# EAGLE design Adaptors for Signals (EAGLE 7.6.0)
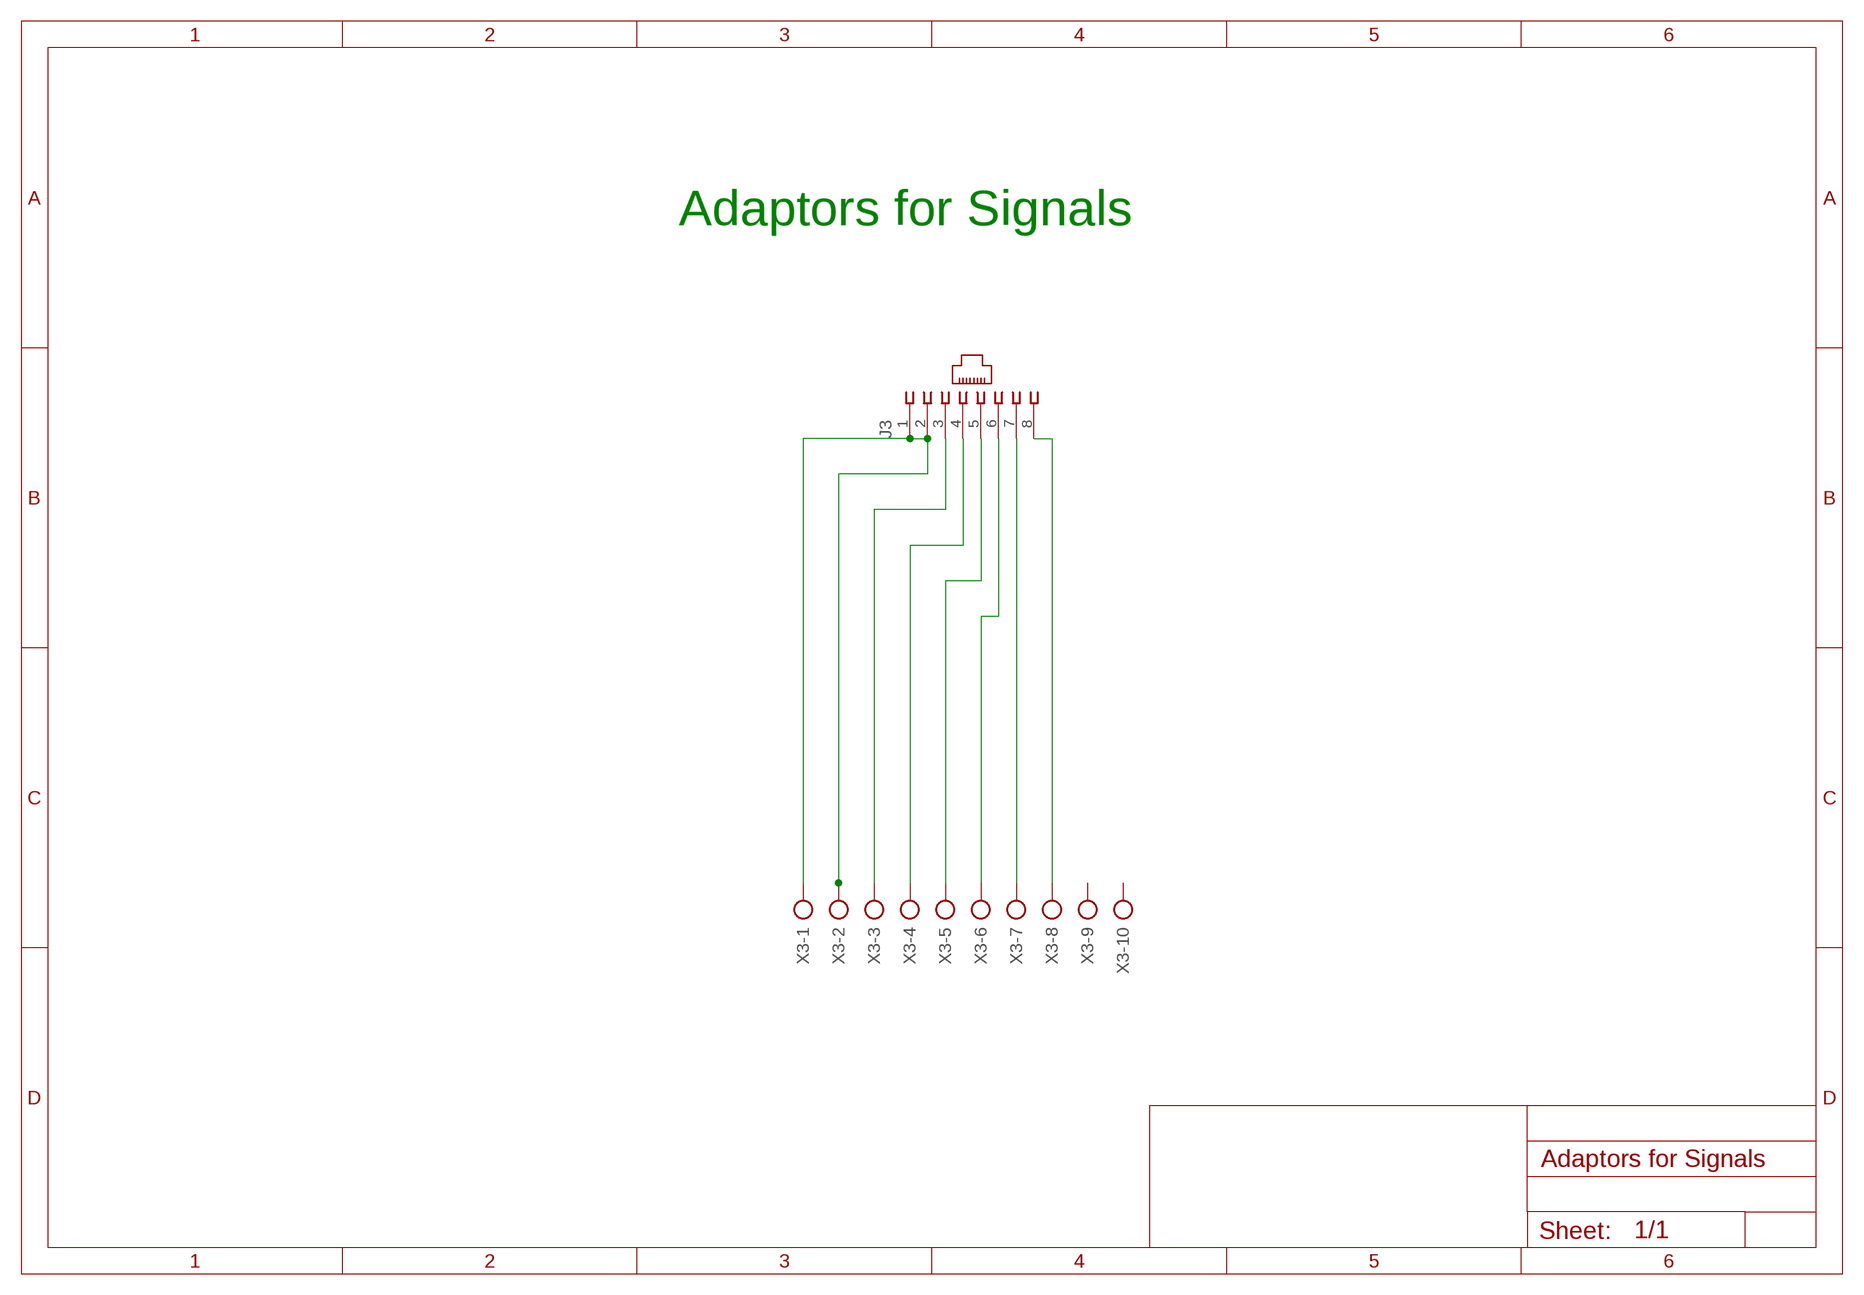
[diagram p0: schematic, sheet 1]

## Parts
J3  520251-4  [520251-4]
X3  AK300/10  [AK300/10]

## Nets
N$1 [Signal]: J3.1 J3.2 X3.1 X3.2
N$2 [Signal]: J3.7 X3.7
N$3 [Signal]: J3.3 X3.3
N$4 [Signal]: J3.4 X3.4
N$5 [Signal]: J3.5 X3.5
N$6 [Signal]: J3.6 X3.6
N$7 [Signal]: J3.8 X3.8
Unconnected: X3.9 X3.10

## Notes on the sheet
- Adaptors for Signals

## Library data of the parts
J3 = con-amp:520251-4: AMP connector; MF: TYCO ELECTRONICS; MPN: 5520251-4; OC_FARNELL: 1557070; OC_NEWARK: 42K7223
X3 = con-ptr500:AK300/10: CONNECTOR; OC_FARNELL: unknown; OC_NEWARK: unknown

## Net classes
1 Signal: width 0.508 mm, drill 0.508 mm, clearance 0.381 mm

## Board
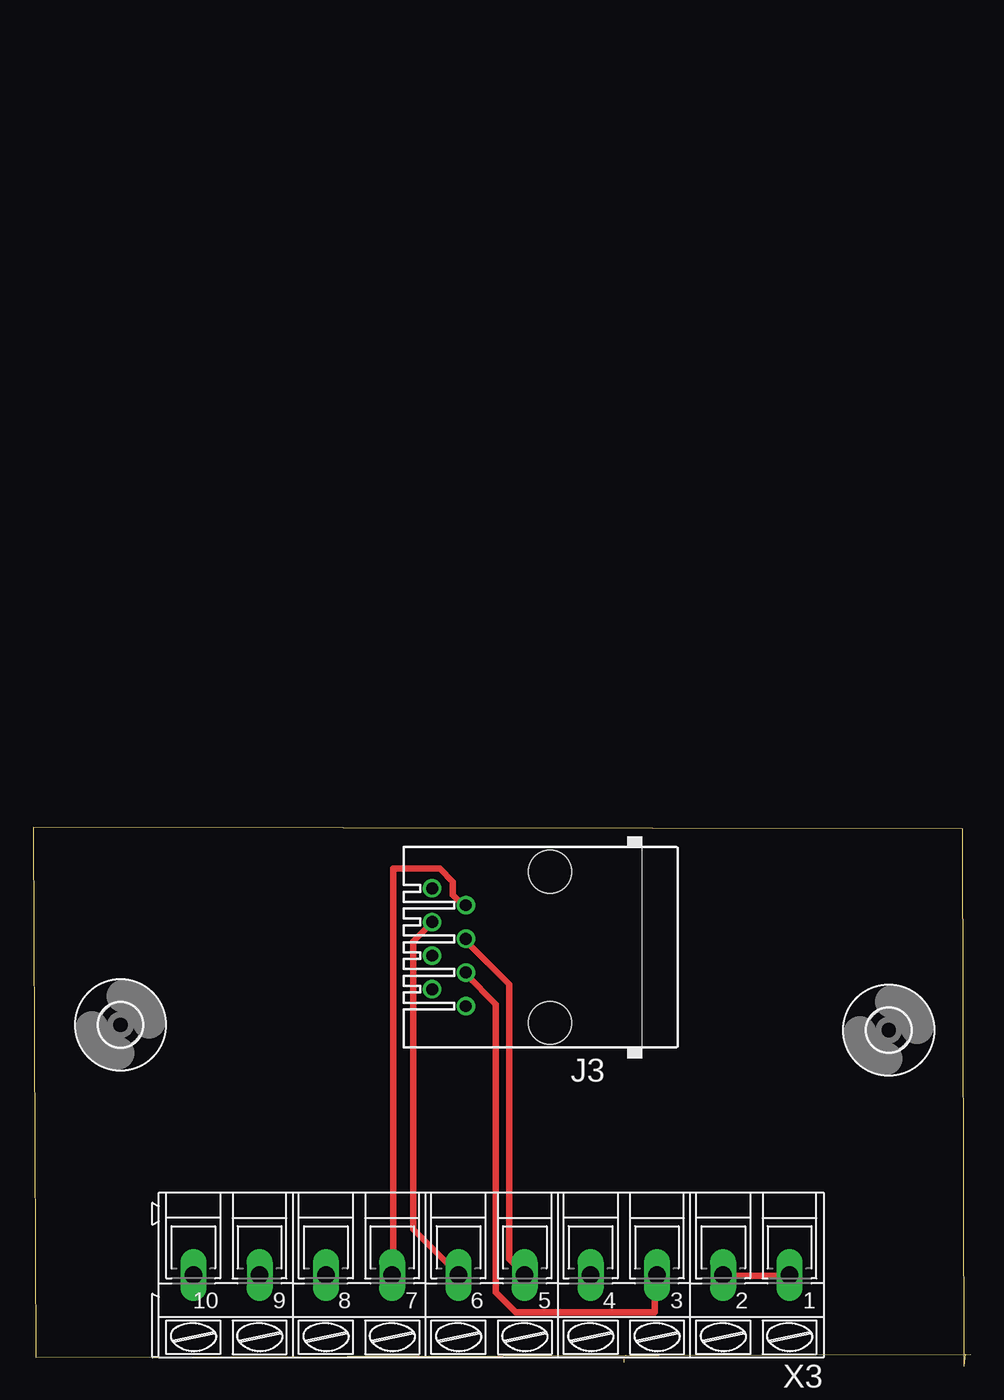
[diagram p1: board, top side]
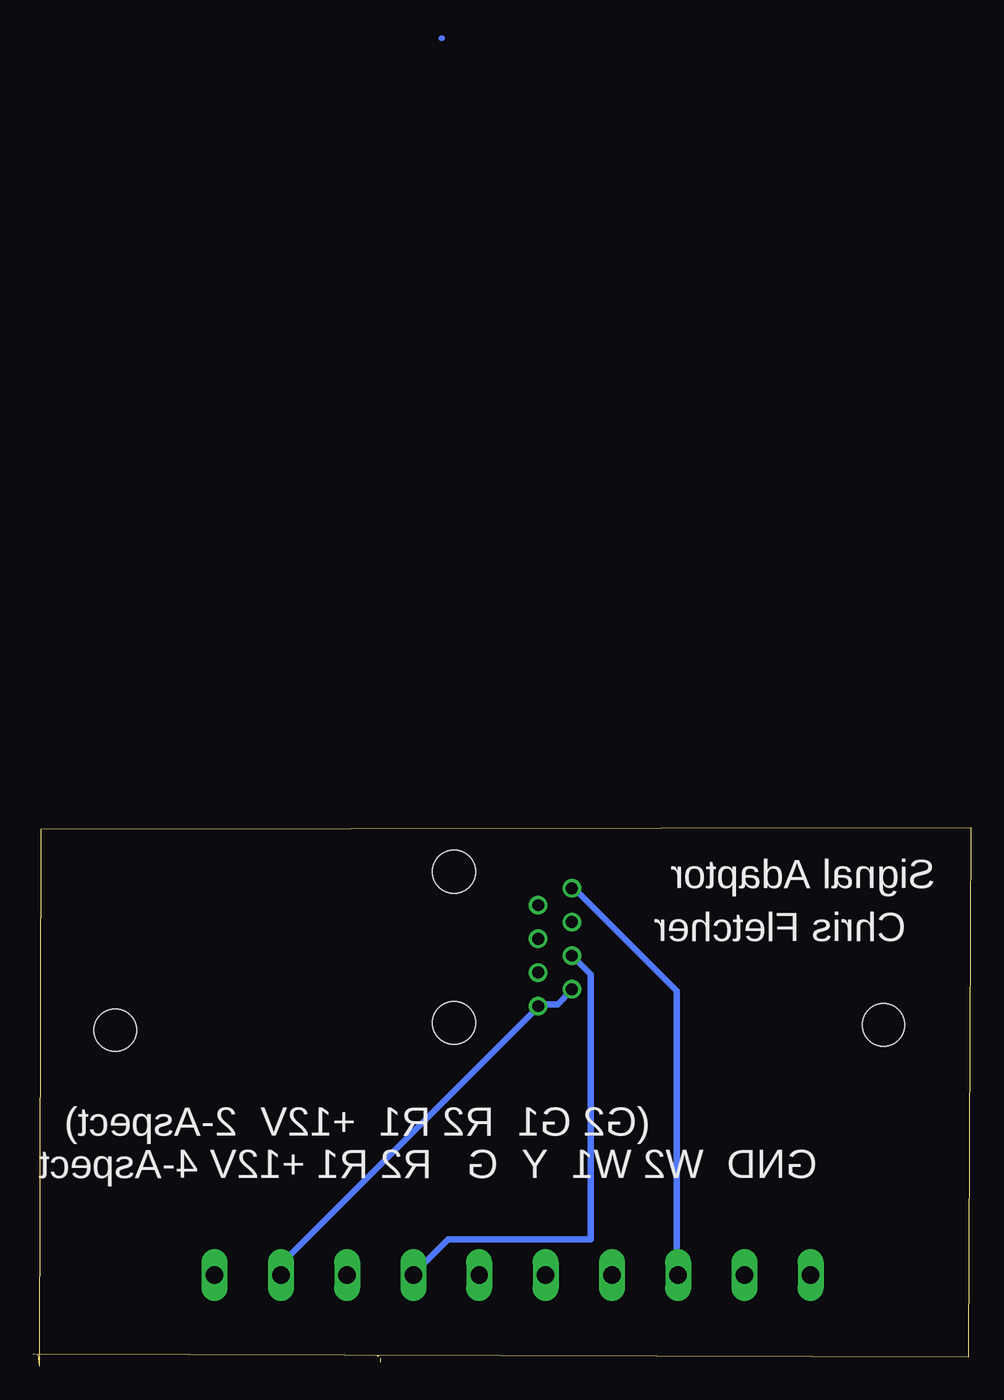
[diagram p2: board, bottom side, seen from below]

Size 70.8 x 40.7 mm. Coordinates in mm from the lower left corner, seen from the top.
Outline: 70.8,0.9 0.2,0.7 0,40.7 70.2,40.6 70.3,0 70.4,0.9
Outline: 44.8,0.8 44.7,0.8
Outline: 44.6,0.6 44.6,0.3
Copper layers (1*16): Top 0.035mm / dielectric 1.5mm / Bottom 0.035mm
Design rules "default": minimum track width 10mil, minimum drill 24mil, track to track 8mil, track to pad 8mil, pad to pad 8mil, via to via 8mil, smd to smd 8mil, copper to edge 40mil, drill to drill 8mil, minimum pad ring 10mil, minimum via ring 8mil, stop-mask expansion 4mil, vias tented up to drill 0mil, thermal gap 10mil

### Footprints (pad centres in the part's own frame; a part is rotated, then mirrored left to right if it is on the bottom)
520251-4 = drill 0.889: 1 -4.445,6.35; 2 -3.175,8.89; 3 -1.905,6.35; 4 -0.635,8.89; 5 0.635,6.35; 6 1.905,8.89; 7 3.175,6.35; 8 4.445,8.89 | hole 3.251: -5.715,0; 5.715,0
3,2 = hole 3.2: 0,0
AK300/10 = drill 1.321 long: 1 -22.504,0; 2 -17.501,0; 3 -12.497,0; 4 -7.493,0; 5 -2.515,0; 6 2.489,0; 7 7.493,0; 8 12.497,0; 9 17.501,0; 10 22.504,0

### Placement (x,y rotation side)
J3  39.02,31.66 90 top
U$1  [3,2]  6.6,25.8 0 top
U$2  [3,2]  64.6,25.4 0 top
X3  34.6,6.9 180 top

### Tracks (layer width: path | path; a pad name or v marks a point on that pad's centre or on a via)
N$1
  Top 0.508: X3.2 52.2,6.85 56.95,6.85 X3.1
  Bottom 0.508: J3.2 30.2,28.35 31.2,27.35 32.45,27.35 J3.1 32.7,27.1 51.95,7.85 51.95,7.1 X3.2
N$2
  Top 0.508: J3.7 32.45,34.85 31.7,35.6 31.7,36.6 30.7,37.6 27.2,37.6 27.2,7.1 X3.7
N$3
  Top 0.508: J3.3 32.7,29.6 34.95,27.35 34.95,5.6 36.45,4.1 46.95,4.1 46.95,6.85 X3.3
N$4
  Bottom 0.508: J3.4 29.95,30.85 28.7,29.6 28.7,9.6 39.45,9.6 41.95,7.1 X3.4
N$5
  Top 0.508: J3.5 32.7,32.1 35.95,28.85 35.95,8.1 36.95,7.1 X3.5
N$6
  Top 0.508: J3.6 29.95,33.35 28.7,32.1 28.7,10.35 31.95,7.1 X3.6
N$7
  Bottom 0.508: J3.8 29.95,36.1 22.2,28.35 22.2,7.1 X3.8
N$29
  Bottom 0.406: 39.9,100.3 40,100.3

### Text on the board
bPlace: Signal Adaptor | Chris Fletcher | (G2 G1 R2 R1 +12V 2-Aspect) | GND W2 W1 Y G R2 R1 +12V 4-Aspect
